TYPE STR_NDI :
STRUCT	
	AV101_OPEN	,	
	AV101_CLOSE	,	
	AV102_OPEN	,	
	AV102_CLOSE	,	
	AV103_OPEN	,
	AV103_CLOSE	,
	AV104_OPEN	,
	AV104_CLOSE	,
	AV105_OPEN	,
	AV105_CLOSE	,
	AV106_OPEN	,
	AV106_CLOSE	,
	CY1_OPEN	,
	CY1_CLOSE	,
	CY2_OPEN	,
	CY2_CLOSE	,
	GV1_OPEN	,
	GV1_CLOSE	,
	Lid_Closed	,
	Water_Leak_Sensor01	,
	Water_Leak_Sensor02	,
	Water_Leak_Sensor03	,
	Water_Leak_Sensor04	,
//	LID_heater_OT	,
//	Chamber_heater_OT	,
	Chiller_Controller_ALM	,
	PG_PS1_Pressure_Switch_Up_Limit	,
	PG_PS1_Pressure_Switch_Down_Limit	,
	MS1_ALM	,
	PS1_Pressure_Switch	,
(*	Forline_Heater1_OT	,
	Forline_Heater2_OT	,
	Forline_Heater3_OT	,
	Forline_Heater4_OT	,
	Forline_Heater5_OT	,
	Forline_Heater6_OT	,
	Forline_Heater7_OT	,
	Forline_Heater8_OT	,
	Turbo_Pump_Heater_OT	,
	Pendulum_Valve_Heater_OT	,
	IGS_Heater_OT	,
	Tape_Heater_OT	,
	Gate_Valve_OT	,
	Stage_Heater_OT	,
*)	CDA_OK	,
	Lift_Pin_Middle1	,
	Lift_Pin_Middle2	,
	FL02B2	,
	FL03B2	,
	FL04B2	,
	AV1		,
	AV2		,
	AV3		,
	AV4		,
	AV26	,
	AV5		,
	Robot_Extend_TO_PM,
	SYS_CDA_OK,
	SYS_N2_OK,
	TM_Lid_Closed:BOOL;
END_STRUCT
END_TYPE
